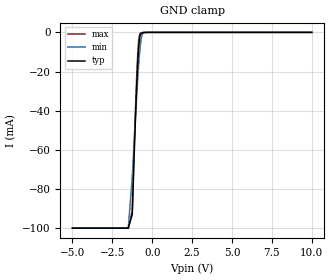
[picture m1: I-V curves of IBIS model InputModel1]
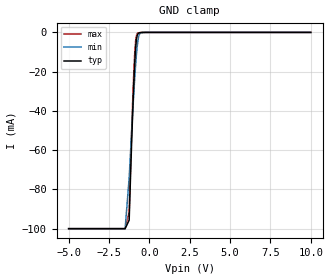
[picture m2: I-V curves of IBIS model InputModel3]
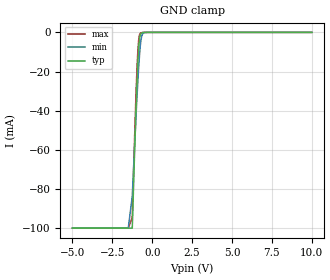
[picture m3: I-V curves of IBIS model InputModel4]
[IBIS Ver]   2.1
[File name]   da016xs5.ibs   | da= SSOP, f016xs= abbr chip name, 5= 5V Vcc
[File Rev]   2.00
[Date]   14-February-96
[Source]   File generated from lab measurements at Intel Corporation
[Notes]   Rev 2.00 All data from actual lab measurements.
[Disclaimer] INTEL DEVELOPER'S SOFTWARE LICENSE AGREEMENT
| BY USING THIS SOFTWARE, YOU ARE AGREEING TO BE BOUND
| BY THE TERMS OFTHIS AGREEMENT.  DO NOT USE THE SOFTWARE
| UNTIL YOU HAVE CAREFULLY READAND AGREED TO THE FOLLOWING
| TERMS AND CONDITIONS.  IF YOU DO NOT AGREETO THE TERMS
| OF THIS AGREEMENT, PROMPTLY RETURN THE SOFTWARE PACKAGE
| ANDANY ACCOMPANYING ITEMS.
| IF YOU USE THIS SOFTWARE, YOU WILL BE BOUND BY THE TERMS
| OF THIS AGREEMENT
| LICENSE: Intel Corporation ("Intel") grants you the non-exclusive right
| to use the enclosed software program ("Software").  You will not use,
| copy, modify, rent, sell or transfer the Software or any portion
| thereof, except as provided in this Agreement.
| System OEM Developers may:
| 1.   Copy the Software for support, backup or archival purposes;
| 2.   Install, use, or distribute Intel owned Software in object code
|   only;
| 3.   Modify and/or use Software source code that Intel directly makes
|   available to you as an OEM Developer;
| 4.   Install, use, modify, distribute, and/or make or have made
|   derivatives ("Derivatives") of Intel owned Software under the
|   terms and conditions in this Agreement, ONLY if you are a System
|   OEM Developer and NOT an end-user.
| RESTRICTIONS:
| YOU WILL NOT:
| 1.   Copy the Software, in whole or in part, except as provided for
|   in this Agreement;
| 2.   Decompile or reverse engineer any Software provided in object
|   code format;
| 3.   Distribute any Software or Derivative code to any end-users,
|   unless approved by Intel in a prior writing.
| TRANSFER: You may transfer the Software to another OEM
| Developer if thereceiving party agrees to the terms of this
| Agreement at the sole risk of any receiving party.
| OWNERSHIP AND COPYRIGHT OF SOFTWARE:
| Title to the Software and all copies thereof remain with Intel
| or its vendors.  The Software iscopyrighted and is protected by
| United States and international copyright laws.  You will not
| remove the copyright notice from the Software.  You agree to
| prevent any unauthorized copying of the Software.
| DERIVATIVE WORK: OEM Developers that make or have made
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[Copyright]   Copyright 1996, Intel Corporation, All Rights Reserved
[Component]   DA28F016XS   | 56-lead SSOP package, 28F016XS
[Manufacturer]  Intel   | Synchronous Flash Memory
|   | operating in 5V Vcc range
[Package]
|Variable   typ   min   max
|The following values apply for the Copper leadframe.
R_pkg   34.81m   20.10m   46.80m
L_pkg   28.00nH   15.75nH   38.77nH
C_pkg   1.09pF   0.68pF   1.50pF
|*****************************Pin Definitions**********************************
[Pin]  signal_name   model_name   R_pin   L_pin   C_pin
  1   CE0#   InputModel1
  2   A12   InputModel1
  3   A13   InputModel1
  4   A14   InputModel3
  5   A15   InputModel1
  6   3/5#   InputModel1
  7   CE1#   InputModel1
  8   NC   InputModel2
  9   A20   InputModel3
 10   A19   InputModel3
 11   A18   InputModel1
 12   A17   InputModel1
 13   A16   InputModel1
 14   VCC   POWER
 15   GND   GND
 16   DQ6   InputOutput
 17   DQ14   InputOutput
 18   DQ7   InputOutput
 19   DQ15   InputOutput
 20   RY/BY#   OpenDrainOutput
 21   OE1#   InputModel1
 22   WE#   InputModel4
 23   WP#   InputModel1
 24   DQ13   InputOutput
 25   DQ5   InputOutput
 26   DQ12   InputOutput
 27   DQ4   InputOutput
 28   VCC   POWER
 29   GND   GND
 30   DQ11   InputOutput
 31   DQ3   InputOutput
 32   DQ10   InputOutput
 33   DQ2   InputOutput
 34   CLK   InputModel5
 35   ADV#   InputModel5
 36   BYTE#   InputModel1
 37   A0   InputModel1
 38   DQ0   InputOutput
 39   DQ8   InputOutput
 40   DQ1   InputOutput
 41   DQ9   InputOutput
 42   VCC   POWER
 43   A8   InputModel1
 44   GND   GND
 45   A7   InputModel1
 46   A6   InputModel1
 47   A5   InputModel1
 48   A4   InputModel1
 49   A3   InputModel1
 50   A2   InputModel1
 51   A1   InputModel1
 52   A9   InputModel1
 53   A10   InputModel1
 54   A11   InputModel1
 55   RP#   InputModel4
 56   VPP   POWER
|**********************Input Model 2************************************
[Model]   InputModel2
Model_type   Input
|   for pin 8(NC)
Vinl = 0.8V
Vinh = 2.0V
| Variable   typ   min   max
C_comp   5.61p   NA   7.6p
[Voltage Range]   5.0V   4.5V   5.5V
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| Models and submodels in the file (7): InputModel1 (Input), InputModel2 (Input), InputModel3 (Input), InputModel4 (Input), InputModel5 (Input), InputOutput (I/O), OpenDrainOutput (Open_drain)
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|**************************Input Model 1***************************************
[Model]   InputModel1
Model_type   Input
|   for pin1(3/5#), CE1#, CE0#, OE#, WP#, BYTE#, A[18:15], A[13:0]
Vinl = 0.8V
Vinh = 2.0V
| Variable   typ   min   max
C_comp   5.61p   NA   7.6p
[Voltage Range]   5.0V   4.5V   5.5V
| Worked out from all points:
|   GND clamp passes 1 mA (typ) near -0.73 V on its own axis
[GND_clamp]
|Voltage I(typ)   I(min)   I(max)
-5V       -99.95mA   -99.95mA   -99.95mA
-1.5V     -99.95mA   -99.95mA   -99.95mA
-1.25V    -92.96mA   -74.04mA   -90.95mA
-1.1V     -55.65mA   -51.01mA   -51.19mA
-1V       -33.11mA   -36.32mA   -27.73mA
-950mV    -23.17mA   -29.39mA   -17.78mA
-900mV    -14.53mA   -22.64mA   -9.695mA
-850mV    -7.833mA   -16.49mA   -4.184mA
-750mV    -1.35mA    -7.041mA   -521.9uA
-650mV    -265.4uA   -1.784mA   -152.7uA
-500mV    -44.52uA   -116.6uA   -16.83uA
10V       0A         0A         0A
[POWER_clamp]
| Input buffer circuits of this product do not intrinsically
| require a [POWER_clamp] definition.  This zero current
| [POWER_clamp] is provided for compatibility with some ibis
| parsers.
|   Voltage  I(typ)   I(min)   I(max)
-5V       0A         0A         0A
-4.75V    0A         0A         0A
9.75V     0A         0A         0A
10V       0A         0A         0A
|*********************Input Model 3**************************************
[Model]   InputModel3
Model_type   Input
|   for A[20], A[19], A[14]
Vinl = 0.8V
Vinh = 2.0V
| Variable   typ   min   max
C_comp   5.61p   NA   7.6p
[Voltage Range]   5.0V   4.5V   5.5V
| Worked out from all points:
|   GND clamp passes 1 mA (typ) near -0.72 V on its own axis
[GND_clamp]
|Voltage I(typ)   I(min)   I(max)
-5V       -99.95mA   -99.95mA   -99.95mA
-1.5V     -99.95mA   -99.95mA   -99.95mA
-1.25V    -95.61mA   -74.11mA   -91.28mA
-1.1V     -56.86mA   -50.87mA   -51mA
-1V       -33.64mA   -36.12mA   -27.59mA
-950mV    -23.47mA   -29.17mA   -17.64mA
-900mV    -14.69mA   -22.58mA   -9.632mA
-850mV    -7.929mA   -16.55mA   -4.193mA
-750mV    -1.418mA   -6.928mA   -582.8uA
-650mV    -309.5uA   -1.797mA   -190.1uA
-500mV    -55.99uA   -137.2uA   -23.18uA
10V       0A         0A         0A
[POWER_clamp]
| Input buffer circuits of this product do not intrinsically
| require a [POWER_clamp] definition.  This zero current
| [POWER_clamp] is provided for compatibility with some ibis
| parsers.
|   Voltage  I(typ)   I(min)   I(max)
-5V       0A         0A         0A
-4.75V    0A         0A         0A
9.75V     0A         0A         0A
10V       0A         0A         0A
|**********************Input Model 4***************************************
[Model]   InputModel4
Model_type   Input
|   for RP#, WE#
Vinl = 0.8V
Vinh = 2.0V
| Variable   typ   min   max
C_comp   5.61p   NA   7.6p
[Voltage Range]   5.0V   4.5V   5.5V
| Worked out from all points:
|   GND clamp passes 1 mA (typ) near -0.73 V on its own axis
[GND_clamp]
|Voltage I(typ)   I(min)   I(max)
-5V       -99.95mA   -99.95mA   -99.95mA
-1.5V     -99.95mA   -99.95mA   -99.95mA
-1.25V    -99.95mA   -83.71mA   -94.58mA
-1.1V     -60.17mA   -57.48mA   -52.75mA
-1V       -35.39mA   -40.15mA   -28.2mA
-950mV    -24.54mA   -32.57mA   -17.85mA
-900mV    -15.18mA   -25.02mA   -9.577mA
-850mV    -8.031mA   -18.13mA   -4.078mA
-750mV    -1.321mA   -7.097mA   -514.4uA
-650mV    -215.8uA   -1.753mA   -148uA
-500mV    -23.9uA    -122.1uA   -15.49uA
10V       0A         0A         0A
[POWER_clamp]
| Input buffer circuits of this product do not intrinsically
| require a [POWER_clamp] definition.  This zero current
| [POWER_clamp] is provided for compatibility with some ibis
| parsers.
|   Voltage  I(typ)   I(min)   I(max)
-5V       0A         0A         0A
-4.75V    0A         0A         0A
9.75V     0A         0A         0A
10V       0A         0A         0A
